(* Logix 5000 AddOnInstructionDefinition export PF_Safety_Diag_KE5; software revision 32.01 *)

ADD_ON_INSTRUCTION PF_Safety_Diag_KE5   (* revision 1.0, vendor Pepperl+Fuchs *)
// Reads diagnostics from a safety monitor on a VBg-EP1-KE5...
VAR_INPUT
   Trigger : BOOL; {visible}
   Safety_Monitor_Address : SINT; {visible}   // The address the safety monitor has been set to. Use 0 for Internal safety monitors
   ASi_Network : SINT; {visible}   // Which AS-i network is mailbox command being sent to. 0/1 is network 1, 2 is network 2
   Object : SINT; {visible}
END_VAR
VAR_OUTPUT
   EN : BOOL; {access Read Only, visible}   // Instruction is enabled
   DN : BOOL; {access Read Only, visible}   // DN bit, When on the instruction has completed. Check ER bit for Error
   ER : BOOL; {access Read Only, visible}   // If the DN bit is on and ER bit is off then command was successful. If ER bit is on then check status byte
END_VAR
VAR_IN_OUT
   ReadStringCmdMSG : MESSAGE; {required}
   ReadStringResponseMSG : MESSAGE; {required}
   Source : SINT[4]; {required}
   Destination : SINT[256]; {required}
END_VAR
VAR_OUTPUT
   State_of_OSSD_1 : SINT; {access Read Only, visible}   // 0 Green 1 Green flashing 2 Yellow 3 Yellow flashing 4 Red 5 Red flashing 6 Grey (OSSD not used) 7 Reserved
   State_of_OSSD_2 : SINT; {access Read Only, visible}   // 0 Green 1 Green flashing 2 Yellow 3 Yellow flashing 4 Red 5 Red flashing 6 Grey (OSSD not used) 7 Reserved
   State_of_OSSD_3 : SINT; {access Read Only, visible}   // 0 Green 1 Green flashing 2 Yellow 3 Yellow flashing 4 Red 5 Red flashing 6 Grey (OSSD not used) 7 Reserved
   State_of_OSSD_4 : SINT; {access Read Only, visible}   // 0 Green 1 Green flashing 2 Yellow 3 Yellow flashing 4 Red 5 Red flashing 6 Grey (OSSD not used) 7 Reserved
   State_of_OSSD_5 : SINT; {access Read Only, visible}   // 0 Green 1 Green flashing 2 Yellow 3 Yellow flashing 4 Red 5 Red flashing 6 Grey (OSSD not used) 7 Reserved
   State_of_OSSD_6 : SINT; {access Read Only, visible}   // 0 Green 1 Green flashing 2 Yellow 3 Yellow flashing 4 Red 5 Red flashing 6 Grey (OSSD not used) 7 Reserved
   State_of_OSSD_7 : SINT; {access Read Only, visible}   // 0 Green 1 Green flashing 2 Yellow 3 Yellow flashing 4 Red 5 Red flashing 6 Grey (OSSD not used) 7 Reserved
   State_of_OSSD_8 : SINT; {access Read Only, visible}   // 0 Green 1 Green flashing 2 Yellow 3 Yellow flashing 4 Red 5 Red flashing 6 Grey (OSSD not used) 7 Reserved
   State_of_OSSD_9 : SINT; {access Read Only, visible}   // 0 Green 1 Green flashing 2 Yellow 3 Yellow flashing 4 Red 5 Red flashing 6 Grey (OSSD not used) 7 Reserved
   State_of_OSSD_10 : SINT; {access Read Only, visible}   // 0 Green 1 Green flashing 2 Yellow 3 Yellow flashing 4 Red 5 Red flashing 6 Grey (OSSD not used) 7 Reserved
   State_of_OSSD_11 : SINT; {access Read Only, visible}   // 0 Green 1 Green flashing 2 Yellow 3 Yellow flashing 4 Red 5 Red flashing 6 Grey (OSSD not used) 7 Reserved
   State_of_OSSD_12 : SINT; {access Read Only, visible}   // 0 Green 1 Green flashing 2 Yellow 3 Yellow flashing 4 Red 5 Red flashing 6 Grey (OSSD not used) 7 Reserved
   State_of_OSSD_13 : SINT; {access Read Only, visible}   // 0 Green 1 Green flashing 2 Yellow 3 Yellow flashing 4 Red 5 Red flashing 6 Grey (OSSD not used) 7 Reserved
   State_of_OSSD_14 : SINT; {access Read Only, visible}   // 0 Green 1 Green flashing 2 Yellow 3 Yellow flashing 4 Red 5 Red flashing 6 Grey (OSSD not used) 7 Reserved
   State_of_OSSD_15 : SINT; {access Read Only, visible}   // 0 Green 1 Green flashing 2 Yellow 3 Yellow flashing 4 Red 5 Red flashing 6 Grey (OSSD not used) 7 Reserved
   State_of_OSSD_16 : SINT; {access Read Only, visible}   // 0 Green 1 Green flashing 2 Yellow 3 Yellow flashing 4 Red 5 Red flashing 6 Grey (OSSD not used) 7 Reserved
END_VAR
VAR_IN_OUT
   Device_Presence : SINT[16]; {required}   // 1 bit for each device object used in safety monitor program
   Index_Colors : SINT[128]; {required}   // An array of diagnostic colors 0 Green 1 Green flashing 2 Yellow 3 Yellow flashing 4 Red 5 Red flashing 6 Gray
END_VAR
VAR_OUTPUT
   Last_Index : DINT; {access Read Only, visible}   // The number of diagnostic indexes returned
   Mode : BOOL; {access Read Only, visible}   // Off=Config Mode, On=Protected mode
   S12 : BOOL; {access Read Only, visible}
   S21 : BOOL; {access Read Only, visible}
   S32 : BOOL; {visible}
   S41 : BOOL; {visible}
   Error_Code : INT; {access Read Only, visible}
END_VAR
VAR
   oneshot : DINT; {access None}
   Null : SINT; {access None}
   Indexcolors : DINT; {access None}
   index0 : DINT; {access None}
   index1 : DINT; {access None}
   Color_Pointer : DINT; {access None}
   watchdog : TIMER := (PRE := 8000); {access None}
END_VAR

ROUTINE Logic   (* ladder *)
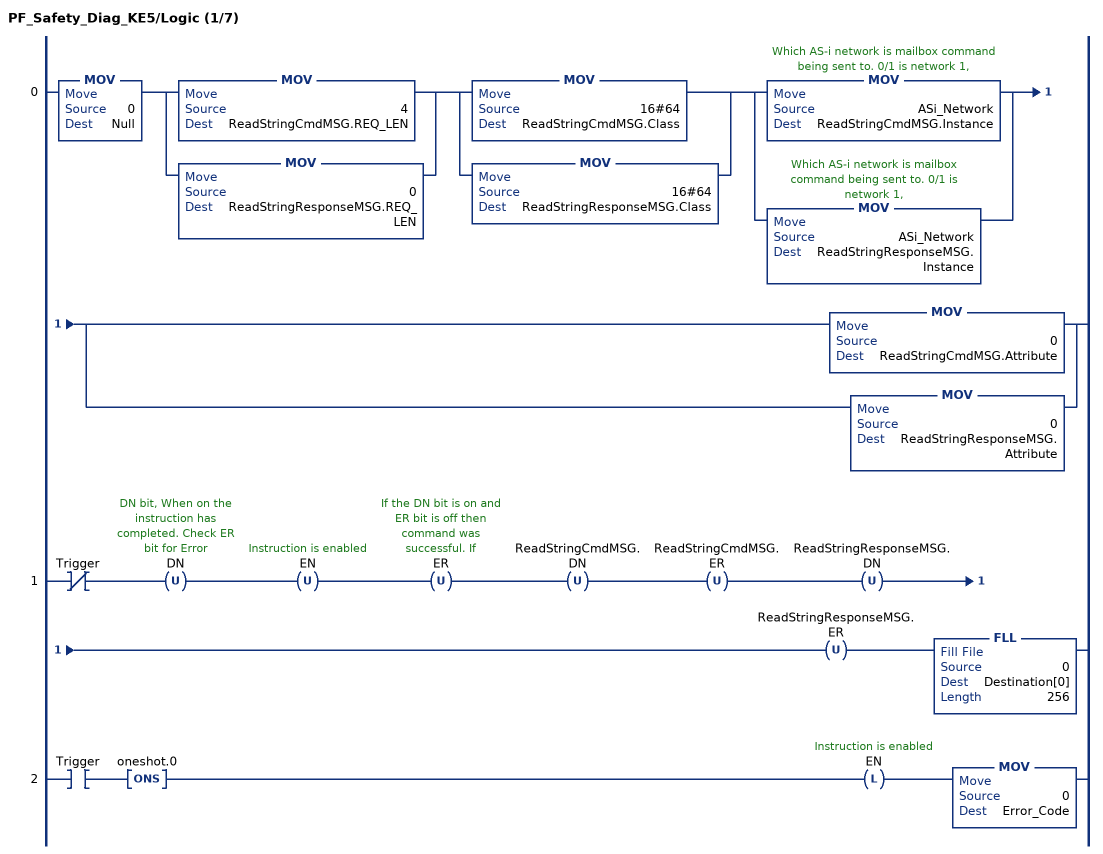
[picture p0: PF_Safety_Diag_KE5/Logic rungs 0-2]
   0: MOV(0,Null)[MOV(4,ReadStringCmdMSG.REQ_LEN) ,MOV(0,ReadStringResponseMSG.REQ_LEN) ][MOV(16#64,ReadStringCmdMSG.Class) ,MOV(16#64,ReadStringResponseMSG.Class) ][MOV(ASi_Network,ReadStringCmdMSG.Instance) ,MOV(ASi_Network,ReadStringResponseMSG.Instance) ][MOV(0,ReadStringCmdMSG.Attribute) ,MOV(0,ReadStringResponseMSG.Attribute) ];
   1: XIO(Trigger)OTU(DN)OTU(EN)OTU(ER)OTU(ReadStringCmdMSG.DN)OTU(ReadStringCmdMSG.ER)OTU(ReadStringResponseMSG.DN)OTU(ReadStringResponseMSG.ER)FLL(0,Destination[0],256);
   2: XIC(Trigger)ONS(oneshot.0)OTL(EN)MOV(0,Error_Code);
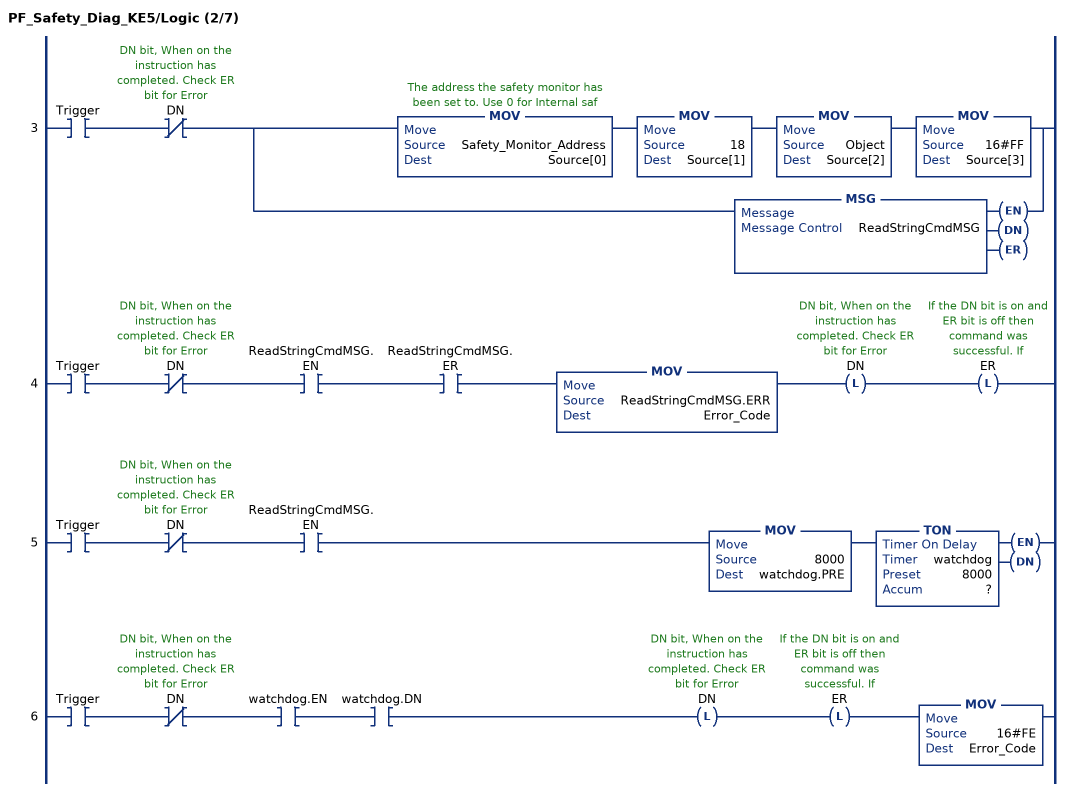
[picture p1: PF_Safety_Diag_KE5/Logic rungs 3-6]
   3: XIC(Trigger)XIO(DN)[MOV(Safety_Monitor_Address,Source[0]) MOV(18,Source[1]) MOV(Object,Source[2]) MOV(16#FF,Source[3]) ,MSG(ReadStringCmdMSG) ];
   4: XIC(Trigger)XIO(DN)XIC(ReadStringCmdMSG.EN)XIC(ReadStringCmdMSG.ER)MOV(ReadStringCmdMSG.ERR,Error_Code)OTL(DN)OTL(ER);
   5: XIC(Trigger)XIO(DN)XIC(ReadStringCmdMSG.EN)MOV(8000,watchdog.PRE)TON(watchdog,?,?);
   6: XIC(Trigger)XIO(DN)XIC(watchdog.EN)XIC(watchdog.DN)OTL(DN)OTL(ER)MOV(16#FE,Error_Code);
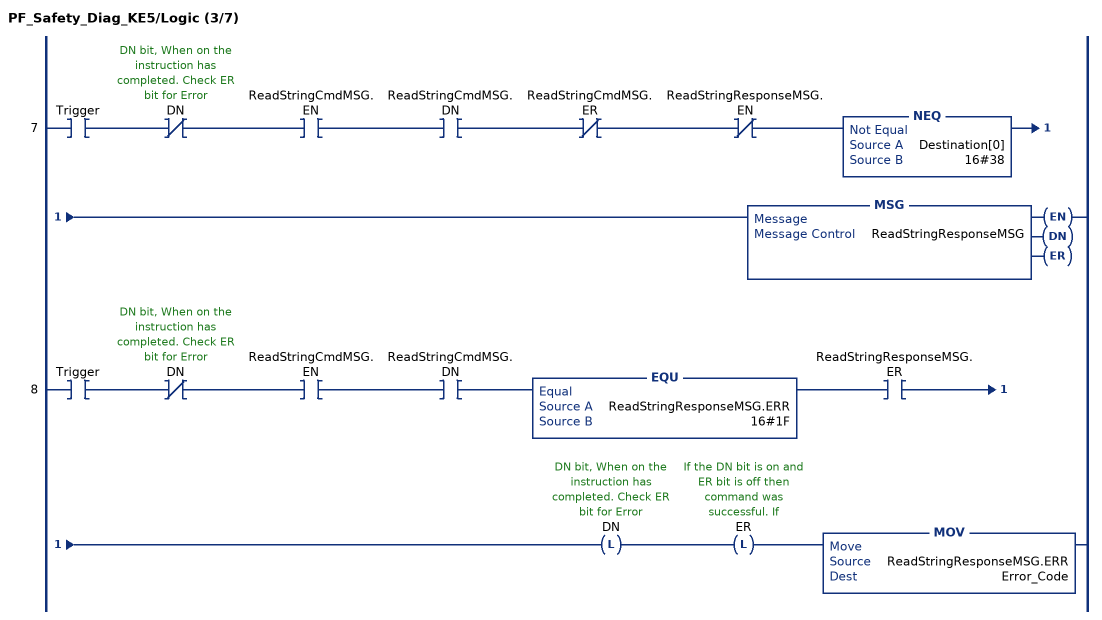
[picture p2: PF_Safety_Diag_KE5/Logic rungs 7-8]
   7: XIC(Trigger)XIO(DN)XIC(ReadStringCmdMSG.EN)XIC(ReadStringCmdMSG.DN)XIO(ReadStringCmdMSG.ER)XIO(ReadStringResponseMSG.EN)NEQ(Destination[0],16#38)MSG(ReadStringResponseMSG);
   8: XIC(Trigger)XIO(DN)XIC(ReadStringCmdMSG.EN)XIC(ReadStringCmdMSG.DN)EQU(ReadStringResponseMSG.ERR,16#1F)XIC(ReadStringResponseMSG.ER)OTL(DN)OTL(ER)MOV(ReadStringResponseMSG.ERR,Error_Code);
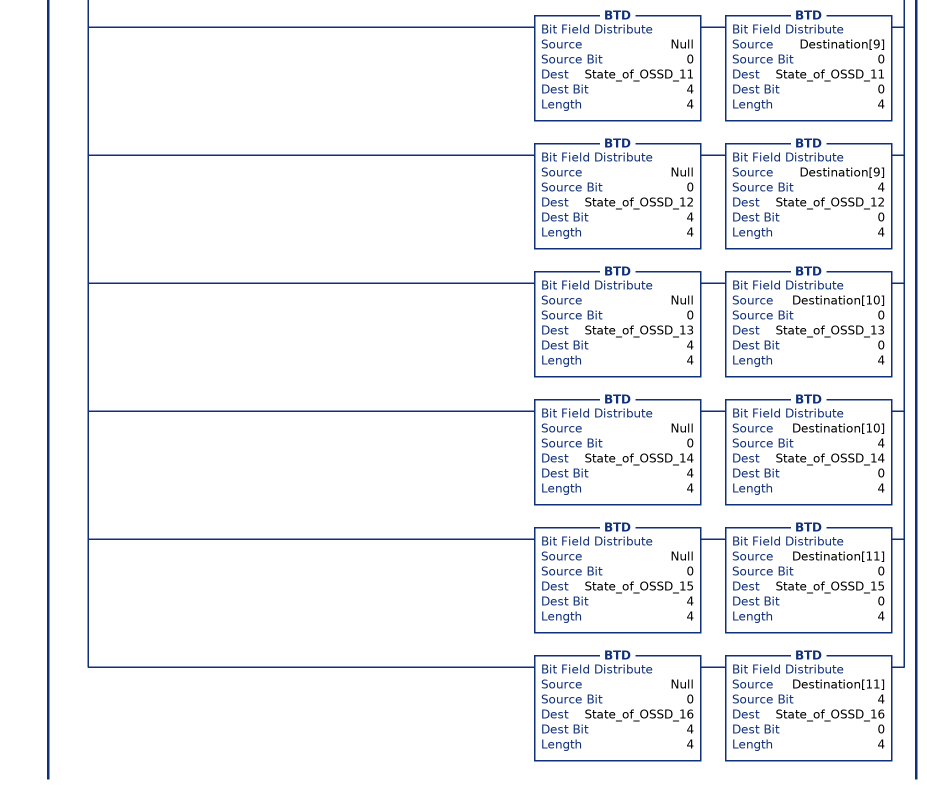
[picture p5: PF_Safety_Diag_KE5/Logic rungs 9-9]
   9: XIC(Trigger)XIO(DN)XIC(ReadStringResponseMSG.DN)XIO(ReadStringResponseMSG.ER)EQU(Destination[0],16#38)ONS(oneshot.2)[[XIC(Destination[3].0) OTL(Mode) ,XIO(Destination[3].0) OTU(Mode) ,XIC(Destination[3].4) OTL(S12) ,XIO(Destination[3].4) OTU(S12) ,XIC(Destination[3].5) OTL(S21) ,XIO(Destination[3].5) OTU(S21) ,XIC(Destination[3].6) OTL(S32) ,XIO(Destination[3].6) OTU(S32) ,XIC(Destination[3].7) OTL(S41) ,XIO(Destination[3].7) OTU(S41) ] ,BTD(Null,0,State_of_OSSD_1,4,4) BTD(Destination[4],0,State_of_OSSD_1,0,4) ,BTD(Null,0,State_of_OSSD_2,4,4) BTD(Destination[4],4,State_of_OSSD_2,0,4) ,BTD(Null,0,State_of_OSSD_3,4,4) BTD(Destination[5],0,State_of_OSSD_3,0,4) ,BTD(Null,0,State_of_OSSD_4,4,4) BTD(Destination[5],4,State_of_OSSD_4,0,4) ,BTD(Null,0,State_of_OSSD_5,4,4) BTD(Destination[6],0,State_of_OSSD_5,0,4) ,BTD(Null,0,State_of_OSSD_6,4,4) BTD(Destination[6],4,State_of_OSSD_6,0,4) ,BTD(Null,0,State_of_OSSD_7,4,4) BTD(Destination[7],0,State_of_OSSD_7,0,4) ,BTD(Null,0,State_of_OSSD_8,4,4) BTD(Destination[7],4,State_of_OSSD_8,0,4) ,BTD(Null,0,State_of_OSSD_9,4,4) BTD(Destination[8],0,State_of_OSSD_9,0,4) ,BTD(Null,0,State_of_OSSD_10,4,4) BTD(Destination[8],4,State_of_OSSD_10,0,4) ,BTD(Null,0,State_of_OSSD_11,4,4) BTD(Destination[9],0,State_of_OSSD_11,0,4) ,BTD(Null,0,State_of_OSSD_12,4,4) BTD(Destination[9],4,State_of_OSSD_12,0,4) ,BTD(Null,0,State_of_OSSD_13,4,4) BTD(Destination[10],0,State_of_OSSD_13,0,4) ,BTD(Null,0,State_of_OSSD_14,4,4) BTD(Destination[10],4,State_of_OSSD_14,0,4) ,BTD(Null,0,State_of_OSSD_15,4,4) BTD(Destination[11],0,State_of_OSSD_15,0,4) ,BTD(Null,0,State_of_OSSD_16,4,4) BTD(Destination[11],4,State_of_OSSD_16,0,4) ];
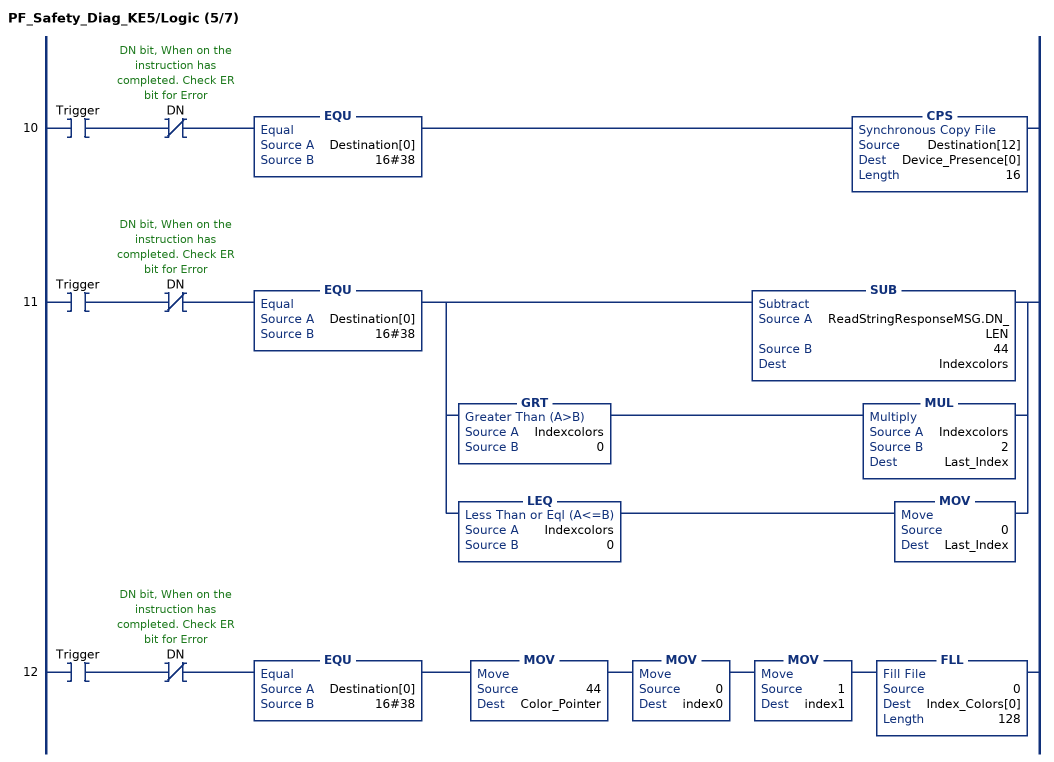
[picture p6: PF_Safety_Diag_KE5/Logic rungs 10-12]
   10: XIC(Trigger)XIO(DN)EQU(Destination[0],16#38)CPS(Destination[12],Device_Presence[0],16);
   11: XIC(Trigger)XIO(DN)EQU(Destination[0],16#38)[SUB(ReadStringResponseMSG.DN_LEN,44,Indexcolors) ,GRT(Indexcolors,0) MUL(Indexcolors,2,Last_Index) ,LEQ(Indexcolors,0) MOV(0,Last_Index) ];
   12: XIC(Trigger)XIO(DN)EQU(Destination[0],16#38)MOV(44,Color_Pointer)MOV(0,index0)MOV(1,index1)FLL(0,Index_Colors[0],128);
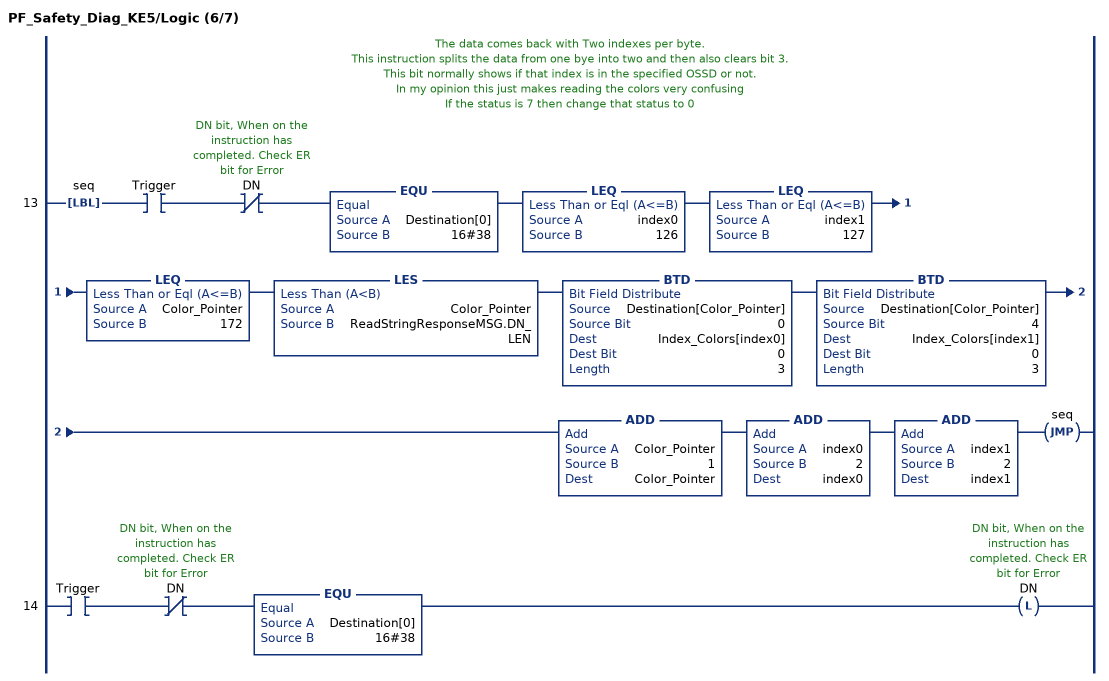
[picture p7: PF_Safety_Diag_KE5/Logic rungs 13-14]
   // The data comes back with Two indexes per byte.
   // This instruction splits the data from one bye into two and then also clears bit 3.
   // This bit normally shows if that index is in the specified OSSD or not.
   // In my opinion this just makes reading the colors very confusing
   // If the status is 7 then change that status to 0
   13: LBL(seq)XIC(Trigger)XIO(DN)EQU(Destination[0],16#38)LEQ(index0,126)LEQ(index1,127)LEQ(Color_Pointer,172)LES(Color_Pointer,ReadStringResponseMSG.DN_LEN)BTD(Destination[Color_Pointer],0,Index_Colors[index0],0,3)BTD(Destination[Color_Pointer],4,Index_Colors[index1],0,3)ADD(Color_Pointer,1,Color_Pointer)ADD(index0,2,index0)ADD(index1,2,index1)JMP(seq);
   14: XIC(Trigger)XIO(DN)EQU(Destination[0],16#38)OTL(DN);
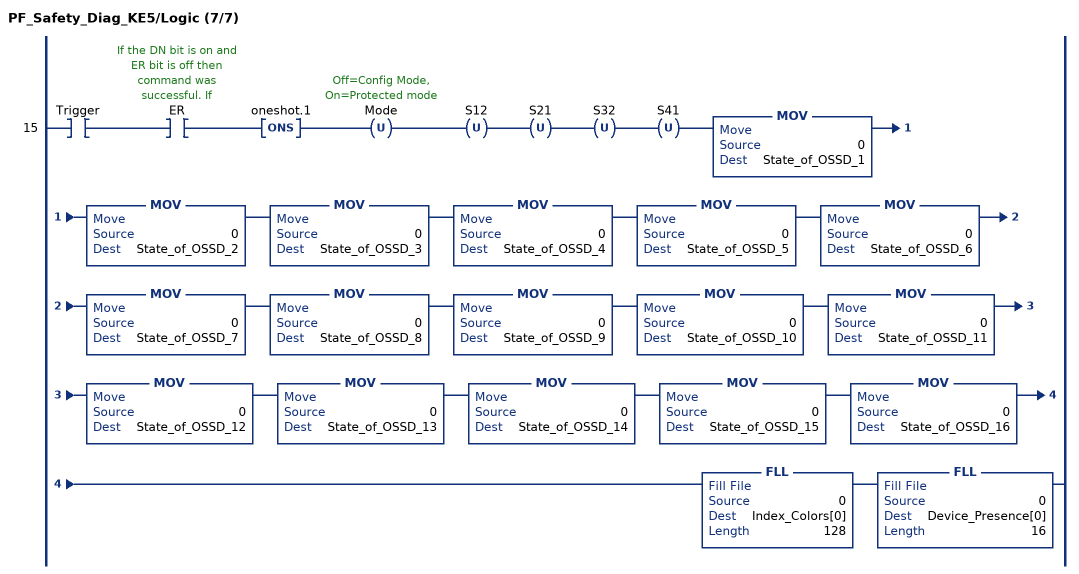
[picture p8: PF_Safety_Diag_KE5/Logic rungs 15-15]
   15: XIC(Trigger)XIC(ER)ONS(oneshot.1)OTU(Mode)OTU(S12)OTU(S21)OTU(S32)OTU(S41)MOV(0,State_of_OSSD_1)MOV(0,State_of_OSSD_2)MOV(0,State_of_OSSD_3)MOV(0,State_of_OSSD_4)MOV(0,State_of_OSSD_5)MOV(0,State_of_OSSD_6)MOV(0,State_of_OSSD_7)MOV(0,State_of_OSSD_8)MOV(0,State_of_OSSD_9)MOV(0,State_of_OSSD_10)MOV(0,State_of_OSSD_11)MOV(0,State_of_OSSD_12)MOV(0,State_of_OSSD_13)MOV(0,State_of_OSSD_14)MOV(0,State_of_OSSD_15)MOV(0,State_of_OSSD_16)FLL(0,Index_Colors[0],128)FLL(0,Device_Presence[0],16);
END_ROUTINE
END_ADD_ON_INSTRUCTION
